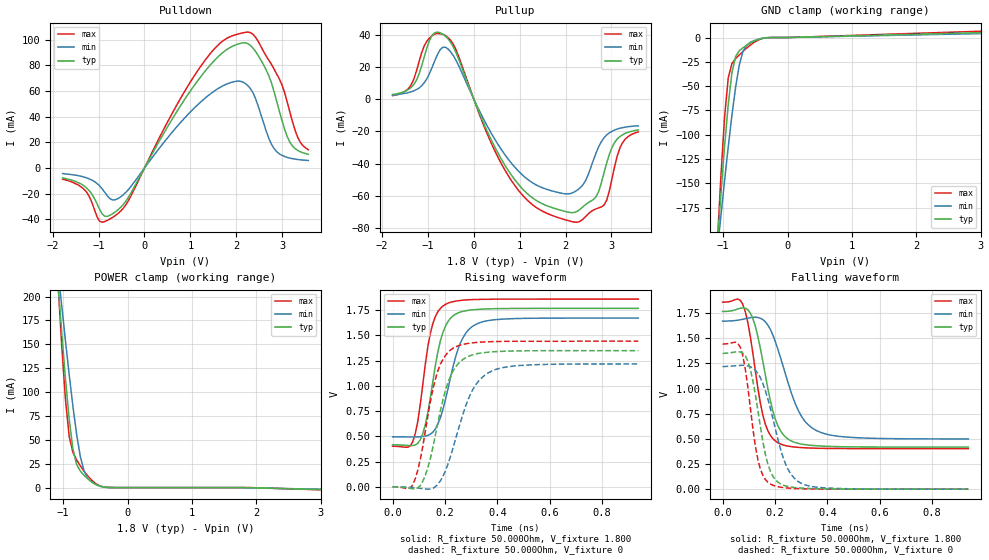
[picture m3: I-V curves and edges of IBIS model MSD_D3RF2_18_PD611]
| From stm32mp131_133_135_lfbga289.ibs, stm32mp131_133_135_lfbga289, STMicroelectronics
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[Model] MSD_D3RF2_18_PD611
Model_type   I/O
C_comp 2.419pF   2.337pF   2.541pF
Vinh = 1.150V
Vinl = 650.000mV
Vmeas = 900.000mV
Vref = 900.000mV
[Model Spec]
Vinh   1.150V   1.100V   1.200V
Vinl   650.000mV   600.000mV   700.000mV
Vmeas   900.000mV   850.000mV   950.000mV
Vref   900.000mV   850.000mV   950.000mV
[Temperature Range]   25.000   125.000   -40.000
[Voltage Range]   1.800V   1.700V   1.900V
[GND Clamp Reference]   0.00V   0.00V   0.00V
[Pulldown Reference]   0.00V   0.00V   0.00V
[POWER Clamp Reference]   1.800V   1.700V   1.900V
[Pullup Reference]   1.800V   1.700V   1.900V
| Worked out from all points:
|   slope of the pulldown table from 0 to 0.27 V, typ, clamps not added: 15.3 ohm
|   slope of the pullup table from 0 to 0.27 V, typ, clamps not added: 14.6 ohm
|   GND clamp passes 1 mA (typ) near -0.40 V on its own axis
|   POWER clamp passes 1 mA (typ) near -0.41 V on its own axis
|   rising waveform, R_fixture 50.000Ohm, V_fixture 1.800: 20-80 % time 57.7ps typ, 73.1ps min, 50.2ps max; typ from 0.418 V to 1.77 V
|   rising waveform, R_fixture 50.000Ohm, V_fixture 0: 20-80 % time 75.3ps typ, 95ps min, 66.5ps max; typ from 0.001 V to 1.35 V
|   falling waveform, R_fixture 50.000Ohm, V_fixture 1.800: 20-80 % time 66ps typ, 93.9ps min, 55.7ps max; typ from 1.77 V to 0.418 V
|   falling waveform, R_fixture 50.000Ohm, V_fixture 0: 20-80 % time 55.5ps typ, 77.8ps min, 46.2ps max; typ from 1.35 V to 0 V
[GND Clamp]
-1.785V   -902.8mA   -690.1mA   -1.212A
-1.094V   -215.3mA   -221.5mA   -216.2mA
-1.036V   -162.4mA   -184.2mA   -144.2mA
-978.8mV  -112.7mA   -147.8mA   -82.77mA
-921.2mV  -69.01mA   -112.7mA   -41.62mA
-863.6mV  -36.19mA   -80mA      -26.75mA
-806.1mV  -19.39mA   -50.94mA   -21.76mA
-748.5mV  -13.55mA   -28.08mA   -17.89mA
-690.9mV  -10.49mA   -14.03mA   -14.25mA
-575.8mV  -5.7mA     -4.889mA   -7.701mA
-287.9mV  -76.48uA   -127.3uA   -62uA
3.57V     6.005mA    4.786mA    7.679mA
[Power Clamp]
-1.77V    884.1mA    691.1mA    1.161A
-1.079V   213.2mA    227.1mA    213.1mA
-1.021V   161.5mA    189.8mA    147.5mA
-963.6mV  113.5mA    153.4mA    91.67mA
-906.1mV  71.67mA    118.2mA    53.57mA
-848.5mV  40.47mA    85.14mA    36.75mA
-790.9mV  24.17mA    55.75mA    28.98mA
-733.3mV  17.3mA     32.49mA    22.73mA
-618.2mV  9.163mA    9.916mA    12.2mA
-503mV    3.524mA    3.614mA    4.591mA
-272.7mV  32uA       104.5uA    32.1uA
3.585V    -3.042mA   -2.585mA   -3.657mA
[Pulldown]
-1.785V   -7.8mA     -4.3mA     -8.7mA
-1.267V   -15.3mA    -7.6mA     -18.5mA
-978.8mV  -32.1mA    -13.9mA    -41.41mA
-575.8mV  -32.49mA   -23.76mA   -35.41mA
1.267V    73.04mA    52.77mA    81.35mA
1.727V    90.57mA    64.39mA    99.47mA
2.245V    97mA       64.46mA    105.9mA
2.591V    80.66mA    35.6mA     91.02mA
2.821V    59.8mA     15.3mA     77.22mA
3.167V    20.2mA     7.7mA      43.7mA
3.339V    13.7mA     6.6mA      23.9mA
3.57V     10.7mA     5.9mA      14.2mA
[Pullup]
-1.77V    2.9mA      2.474mA    2.179mA
-1.367V   7.2mA      4.495mA    8.716mA
-1.136V   20.6mA     8.279mA    28.74mA
-906.1mV  39.67mA    19.85mA    39.33mA
-618.2mV  38.98mA    32.14mA    39.33mA
878.8mV   -49.38mA   -41.65mA   -52.88mA
1.455V    -64.25mA   -54.44mA   -68.75mA
2.203V    -70.07mA   -57.29mA   -76.21mA
2.664V    -60.5mA    -33.36mA   -67.94mA
2.836V    -45.7mA    -23.98mA   -65.61mA
3.182V    -23.2mA    -18.03mA   -30.35mA
3.585V    -19.1mA    -16.6mA    -20.3mA
[Ramp]
R_load=50.000Ohm
dV/dt_r   809.640mV/67.000ps  717.269mV/85.000ps  869.790mV/58.500ps
dV/dt_f   809.640mV/61.500ps  717.269mV/86.500ps  869.790mV/51.500ps
[Rising waveform]
R_fixture=50.000Ohm
V_fixture=1.800
V_fixture_min=1.700
V_fixture_max=1.900
0s        417.5mV    496.3mV    402.8mV
68ps      409.2mV    494.5mV    407.2mV
87ps      415.5mV    494.9mV    530.8mV
106ps     468.2mV    497.2mV    821.9mV
144ps     880mV      522.2mV    1.519V
173ps     1.339V     621.1mV    1.735V
202ps     1.592V     866.1mV    1.808V
259ps     1.732V     1.426V     1.846V
326ps     1.758V     1.619V     1.856V
938ps     1.768V     1.672V     1.86V
[Rising waveform]
R_fixture=50.000Ohm
V_fixture=0
0s        1.095mV    995.2uV    968.6uV
77ps      -18.76mV   -6.222mV   20.18mV
115ps     53.89mV    -17.54mV   397.1mV
144ps     279.7mV    -20.72mV   841.3mV
173ps     636mV      26.23mV    1.15V
202ps     958.3mV    161.3mV    1.302V
230ps     1.144V     379mV      1.372V
307ps     1.309V     967.3mV    1.427V
384ps     1.338V     1.153V     1.439V
938ps     1.349V     1.218V     1.443V
[Falling waveform]
R_fixture=50.000Ohm
V_fixture=1.800
V_fixture_min=1.700
V_fixture_max=1.900
0s        1.766V     1.67V      1.858V
68ps      1.798V     1.683V     1.876V
87ps      1.798V     1.694V     1.761V
106ps     1.75V      1.704V     1.515V
154ps     1.266V     1.684V     732.7mV
183ps     871.5mV    1.585V     531.7mV
211ps     631.3mV    1.391V     461.9mV
288ps     455.1mV    787.4mV    415.6mV
365ps     430.2mV    574.1mV    406.3mV
938ps     418.4mV    498.8mV    403mV
[Falling waveform]
R_fixture=50.000Ohm
V_fixture=0
0s        1.349V     1.218V     1.442V
68ps      1.363V     1.23V      1.409V
96ps      1.275V     1.225V     1.022V
115ps     1.085V     1.204V     616mV
135ps     779.1mV    1.15V      289.3mV
163ps     350.4mV    981.8mV    97.69mV
183ps     175.4mV    797.2mV    50.6mV
240ps     32.59mV    252.6mV    13.5mV
307ps     10.06mV    50.19mV    3.786mV
938ps     2.864uV    36.53uV    0V
